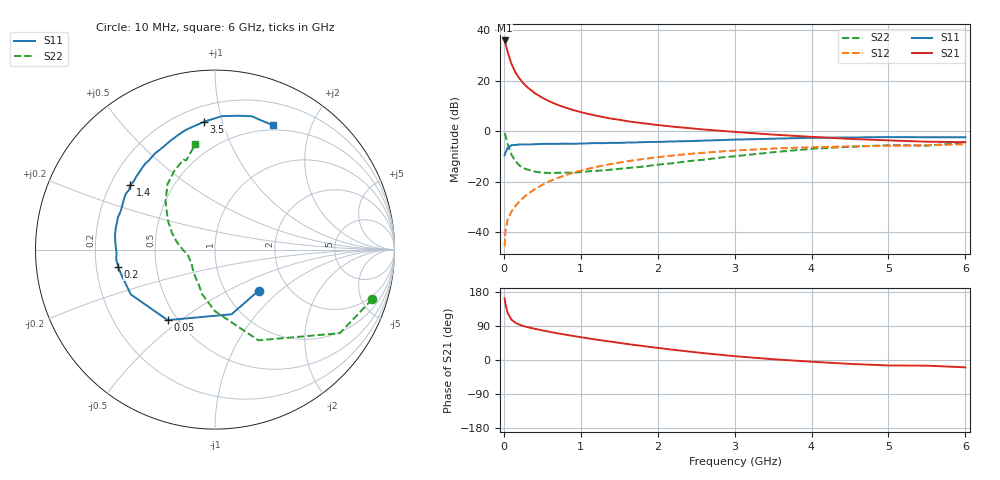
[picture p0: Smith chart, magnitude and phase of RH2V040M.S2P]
! SIEMENS Small Signal Semiconductors
! BFR106
! Si NPN RF Bipolar Junction Transistor in SOT23
! VCE = 2 V  IC = 40 mA
! Common Emitter S-Parameters:  August  1996
# GHz  S  MA  R  50
!  f  S11  S21  S12  S22
! GHz  MAG  ANG  MAG  ANG  MAG  ANG  MAG  ANG
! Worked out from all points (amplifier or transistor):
!   36 points, 10 MHz to 6 GHz, reference 50 ohm
!   highest |S21| = 36.0 dB at 10 MHz (marker M1)
!   |S21| within 3 dB of that: start of sweep to 36.52 MHz
!   unconditionally stable (mu >= 1): 251.3 MHz to 2.663 GHz; 5.136 GHz to end of sweep
!   at 250 MHz: K = 1.00, MSG = 22.8 dB, |S12| = -26.4 dB
!   at 1.4 GHz: K = 1.06, MAG = 7.5 dB, |S12| = -12.9 dB
!   at 6 GHz: K = 1.01, MAG = -0.3 dB, |S12| = -5.1 dB
!   S11 on the Smith chart (normalised r, x): 10 MHz: 1.42, -0.73; 50 MHz: 0.44, -0.45; 200 MHz: 0.29, -0.08; 1.4 GHz: 0.28, +0.31; 3.5 GHz: 0.30, +0.87; 6 GHz: 0.44, +1.47
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0.01  0.334 -43.1  63.4 162.9  0.0053 79.4  0.918 -17.6
0.02  0.3719 -75.7  56.59 149.1  0.0101 69.6  0.8373 -33.8
0.05  0.4734 -123.9  37.14 123.5  0.018 57.2  0.5603 -64.4
0.1  0.531 -151.9  21.63 106.3  0.026 57.6  0.3423 -90.2
0.15  0.5383 -163.7  14.85 98.2  0.033 61.3  0.2587 -106.1
0.2  0.549 -170.0  11.34 93.5  0.0405 64.6  0.2124 -115.6
0.25  0.5529 -174.7  9.088 89.7  0.0478 66.2  0.1878 -125.4
0.3  0.5489 -178.0  7.612 87.1  0.0557 67.8  0.176 -131.7
0.4  0.5561 176.4  5.763 82.4  0.0713 69.3  0.1598 -142.4
0.5  0.5631 171.7  4.636 78.2  0.087 69.4  0.1513 -149.6
0.6  0.5658 167.9  3.888 74.1  0.1037 69.0  0.1497 -154.3
0.7  0.5667 164.5  3.358 70.3  0.119 68.2  0.151 -158.6
0.9  0.5674 157.6  2.652 63.5  0.151 65.9  0.1516 -166.4
1.1  0.5795 151.1  2.21 57.0  0.1816 63.2  0.1612 -170.8
1.4  0.5935 142.6  1.784 48.3  0.2264 58.4  0.1747 -178.1
1.7  0.6031 134.3  1.518 39.5  0.268 53.7  0.1934 174.6
2.2  0.6315 122.0  1.239 27.0  0.3328 45.4  0.2336 163.7
2.8  0.6697 108.0  1.032 14.1  0.3971 35.4  0.3003 149.8
3.5  0.7153 94.9  0.863 2.0  0.4565 24.5  0.3857 135.6
4.5  0.7564 80.4  0.71 -10.3  0.503 10.2  0.4948 117.1
5.5  0.7639 69.1  0.624 -14.9  0.5299 1.4  0.5225 107.9
6  0.7641 65.1  0.611 -19.4  0.5568 -5.4  0.5974 100.5
